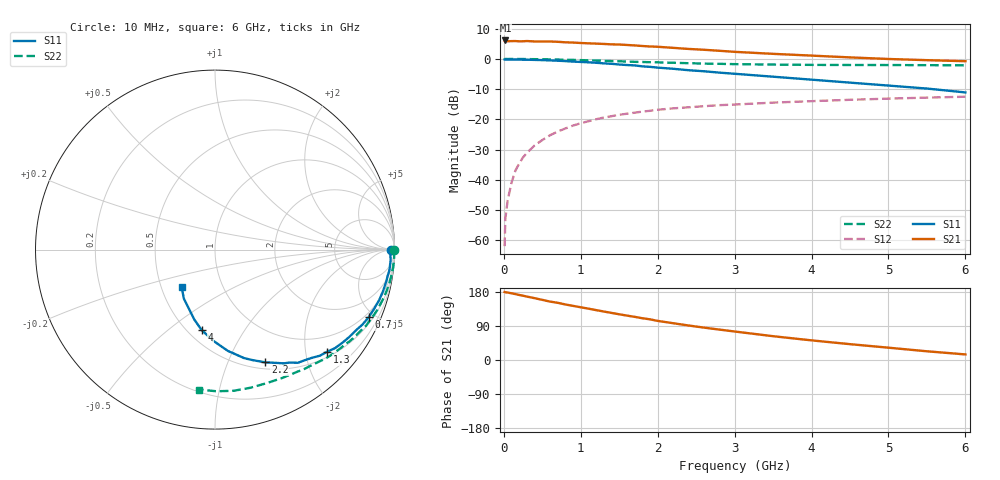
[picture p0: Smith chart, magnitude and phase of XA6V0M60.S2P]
! SIEMENS Discrete & RF Semiconductors
! BFY180
! Si NPN RF Bipolar Junction Transistor in MICRO-X
! VCE = 6 V  IC = 0.6 mA
! Common Emitter S-Parameters:  May  1997
# GHz  S  MA  R  50
!  f  S11  S21  S12  S22
! GHz  MAG  ANG  MAG  ANG  MAG  ANG  MAG  ANG
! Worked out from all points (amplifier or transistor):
!   36 points, 10 MHz to 6 GHz, reference 50 ohm
!   highest |S21| = 6.1 dB at 20 MHz (marker M1)
!   |S21| within 3 dB of that: start of sweep to 2.542 GHz
!   unconditionally stable (mu >= 1): 5.535 GHz to end of sweep
!   at 250 MHz: K = 0.06, MSG = 19.2 dB, |S12| = -32.5 dB
!   at 1.4 GHz: K = 0.40, MSG = 11.9 dB, |S12| = -18.9 dB
!   at 6 GHz: K = 1.01, MAG = 5.1 dB, |S12| = -12.5 dB
!   S11 on the Smith chart (normalised r, x): 10 MHz: 97, -17; 700 MHz: 0.76, -4.63; 1.3 GHz: 0.62, -2.44; 2.2 GHz: 0.58, -1.38; 4 GHz: 0.59, -0.66; 6 GHz: 0.64, -0.29
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0.01  0.9802 -0.2  1.973 179.5  0.0008 70.8  0.9983 -0.2
0.02  0.9791 -0.8  2.023 178.8  0.0023 93.9  0.9999 -0.4
0.05  0.9771 -1.6  1.965 178.1  0.0046 86.7  0.9983 -1.2
0.1  0.9802 -3.4  1.973 176.0  0.009 89.7  0.9991 -2.4
0.15  0.9792 -5.1  1.977 174.0  0.0142 86.7  0.9991 -3.5
0.2  0.9781 -6.9  1.956 171.6  0.0187 85.1  0.9975 -4.7
0.3  0.9713 -10.3  1.979 167.3  0.0279 82.4  0.9945 -7.0
0.4  0.9646 -13.8  1.947 163.2  0.0371 79.5  0.9924 -9.2
0.6  0.946 -20.4  1.946 154.2  0.0546 74.7  0.9827 -13.8
0.7  0.9357 -23.8  1.922 150.9  0.063 71.9  0.9774 -16.0
1.1  0.8799 -36.0  1.813 135.5  0.0933 62.2  0.9489 -24.5
1.3  0.8446 -42.4  1.772 127.9  0.1074 57.7  0.9321 -28.6
1.5  0.809 -48.2  1.732 120.6  0.1192 53.3  0.9153 -32.5
1.7  0.7816 -53.8  1.674 113.9  0.1292 49.8  0.8961 -36.1
2  0.7191 -61.4  1.591 103.2  0.1444 44.7  0.8787 -41.2
2.2  0.6881 -65.9  1.527 97.1  0.1522 41.2  0.8651 -44.5
2.8  0.5945 -78.9  1.366 80.3  0.172 33.3  0.8309 -53.2
3.5  0.5086 -91.0  1.215 62.8  0.1896 25.5  0.8071 -62.5
4  0.4544 -99.4  1.136 51.8  0.2003 20.6  0.7978 -69.0
4.5  0.4057 -106.6  1.061 41.8  0.2111 16.1  0.7945 -75.7
5.5  0.3238 -122.4  0.955 23.0  0.2294 7.3  0.7893 -89.5
6  0.2794 -131.6  0.918 14.7  0.2372 2.7  0.7845 -96.4
